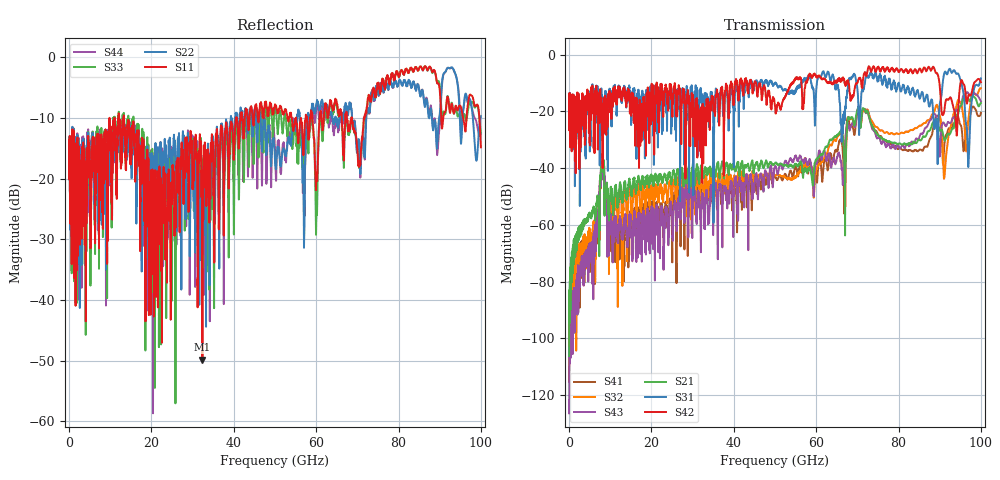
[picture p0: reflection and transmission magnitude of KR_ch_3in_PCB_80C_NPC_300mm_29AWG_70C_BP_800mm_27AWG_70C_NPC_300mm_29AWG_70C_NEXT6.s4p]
# GHz S RI R 45
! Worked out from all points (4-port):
!   4000 points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, 25 MHz to 100 GHz, reference 45 ohm
!   strongest paths, dB at 25 MHz, 25.02 GHz, 50.02 GHz, 75.03 GHz, 100 GHz:
!     S42: -20.0, -17.9, -18.0, -4.4, -9.7
!     S31: -20.0, -21.4, -10.2, -8.7, -8.4
!     S21: -106.2, -44.0, -38.1, -28.3, -17.0
!     S43: -126.4, -57.7, -39.3, -29.4, -16.4
!     S32: -109.4, -52.3, -42.7, -25.9, -11.9
!     S41: -115.3, -68.8, -43.0, -28.1, -20.5
!   lowest |S11| = -49.8 dB at 32.38 GHz (marker M1), VSWR 1.01, Z = 45 + j0.29 ohm
!   |S11| at or under -10 dB: start of sweep to 9.824 GHz; 13.31 GHz to 40.54 GHz (27.23 GHz wide, 101 % of centre); 68.65 GHz to 71.57 GHz (2.921 GHz wide, 4.17 % of centre)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
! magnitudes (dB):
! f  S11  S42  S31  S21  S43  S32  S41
! 25 MHz  -16.1  -20.0  -20.0  -106.2  -126.4  -109.4  -115.3
! 8.05 GHz  -19.6  -23.6  -18.0  -38.5  -36.3  -37.3  -36.5
! 11.72 GHz  -13.5  -13.0  -13.5  -53.6  -62.3  -61.4  -63.0
! 32.38 GHz  -49.8  -23.2  -21.5  -41.8  -49.0  -42.8  -44.6
! 91.25 GHz  -9.0  -18.3  -6.1  -30.2  -24.8  -41.2  -30.2
! 96.85 GHz  -7.7  -15.3  -36.0  -15.2  -13.4  -24.4  -23.8
! 100 GHz  -14.8  -9.7  -8.4  -17.0  -16.4  -11.9  -20.5
